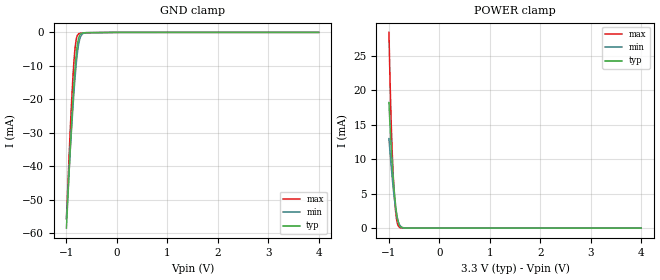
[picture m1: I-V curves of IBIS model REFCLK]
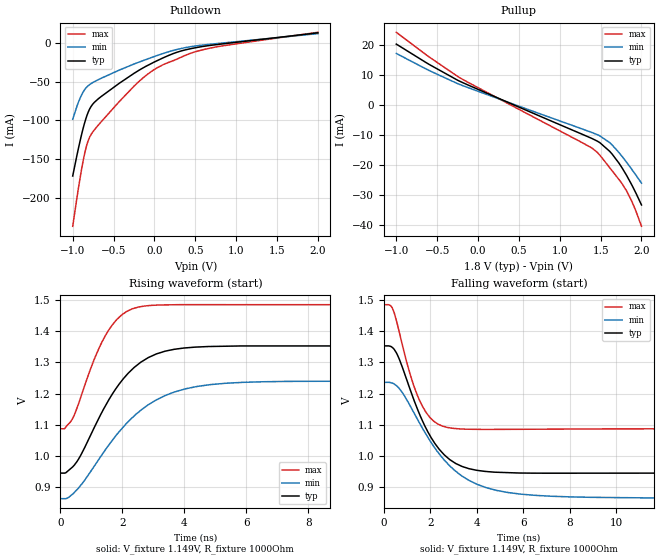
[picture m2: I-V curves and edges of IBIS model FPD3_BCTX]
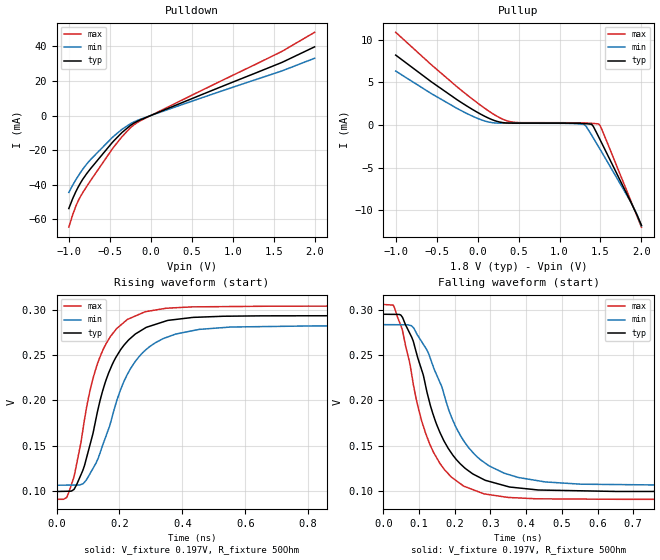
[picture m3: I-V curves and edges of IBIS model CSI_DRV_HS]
|Texas Instruments Incorporated
| Marketing part#   Package-type   #pins
| DS90UB962-Q1   VQFN   64
[IBIS Ver]   4.1
[File name]   ds90ub962q1.ibs
[File Rev]   1.1
[Date]   09/20/2017
[Source]
| Texas Instruments Incorporated.
| 12500 TI Blvd
| Dallas, TX -75243
[Notes]   Revision History:
| Rev 1.2: 09/20/2017
| - Matrix package model added.
| Rev 1.1:  07/22/2016
| - Various signal names modified to reflect the latest datasheet.
| - Various model names modified to reflect I/O character.
| - Unused models removed.
| Rev 1.0: 07/23/2015
| - Initial version of the model
| - Model generated from simulations in TISPICE
| - C_comp although listed in numerical order of value are
|   obtained from varying PVT conditions. For PVT conditions for
|   each specific value refer the buffer description under
|   respective [Model]. IBIS model user is responsible for using
|   appropriate C_comp to simulate for Signal Integrity.
| - Warnings regarding combined Non-monotonicity of various models have been
|   reviewd and considered minor and can be ignored.
| - Model names with a trailing _1p8 contain the model for
|   1.8V operation. Model names with a trailing _3p3 contain the model
|   for 3.3V operation.
[Disclaimer]
| This model is designed as an aid for customers of Texas Instruments.
| TI and its licensors and suppliers make no warranties, either expressed
| or implied, with respect to this  model, including the warranties of
| merchantability or fitness for a particular purpose. The model is
| provided solely on an "as is" basis. The entire risk as to its quality
| and performance is with the customer.
[Copyright]
 (C) Copyright 2015 Texas Instruments Incorporated.All rights reserved.
|   Device
[Component]   DS90UB962-Q1
[Manufacturer]   TI
[Package]  |QFN   64
|   typ   min   max
R_pkg   0   0   0
L_pkg   0   0   0
C_pkg   0   0   0
[Pin]  signal_name   model_name   R_pin   L_pin   C_pin
1   VDD18_P3   POWER   NA   NA   NA
2   VDD18_P2   POWER   NA   NA   NA
3   PDB   PDB   NA   NA   NA
4   TESTEN   IO_LVCMOS   NA   NA   NA
5   REFCLK   REFCLK   NA   NA   NA
6   INTB   IO_OPEN_DRAIN   NA   NA   NA
7   I2C_SDA2   IO_OPEN_DRAIN   NA   NA   NA
8   I2C_SCL2   IO_OPEN_DRAIN   NA   NA   NA
9   GPIO0   IO_LVCMOS   NA   NA   NA
10   GPIO1   IO_LVCMOS   NA   NA   NA
11   I2C_SDA   IO_OPEN_DRAIN   NA   NA   NA
12   I2C_SCL   IO_OPEN_DRAIN   NA   NA   NA
13   VDDL1   POWER   NA   NA   NA
14   GPIO2   IO_LVCMOS   NA   NA   NA
15   GPIO3   IO_LVCMOS   NA   NA   NA
16   VDDIO   POWER   NA   NA   NA
17   GPIO4   IO_LVCMOS   NA   NA   NA
18   GPIO5   IO_LVCMOS   NA   NA   NA
19   GPIO6   IO_LVCMOS   NA   NA   NA
20   GPIO7   IO_LVCMOS   NA   NA   NA
21   VDD_CSI0   POWER   NA   NA   NA
22   CSI0_CLKN   CSI_DRV   NA   NA   NA
23   CSI0_CLKP   CSI_DRV   NA   NA   NA
24   CSI0_D0N   CSI_DRV   NA   NA   NA
25   CSI0_D0P   CSI_DRV   NA   NA   NA
26   CSI0_D1N   CSI_DRV   NA   NA   NA
27   CSI0_D1P   CSI_DRV   NA   NA   NA
28   CSI0_D2N   CSI_DRV   NA   NA   NA
29   CSI0_D2P   CSI_DRV   NA   NA   NA
30   CSI0_D3N   CSI_DRV   NA   NA   NA
31   CSI0_D3P   CSI_DRV   NA   NA   NA
32   VDD18A   POWER   NA   NA   NA
33   VDD_CSI1   POWER   NA   NA   NA
34   CSI1_CLKN   CSI_DRV   NA   NA   NA
35   CSI1_CLKP   CSI_DRV   NA   NA   NA
36   CSI1_D0N   CSI_DRV   NA   NA   NA
37   CSI1_D0P   CSI_DRV   NA   NA   NA
38   CSI1_D1N   CSI_DRV   NA   NA   NA
39   CSI1_D1P   CSI_DRV   NA   NA   NA
40   CSI1_D2N   CSI_DRV   NA   NA   NA
41   CSI1_D2P   CSI_DRV   NA   NA   NA
42   CSI1_D3N   CSI_DRV   NA   NA   NA
43   CSI1_D3P   CSI_DRV   NA   NA   NA
44   VDDL2   POWER   NA   NA   NA
45   MODE   IO_STRAP   NA   NA   NA
46   IDX   IO_STRAP   NA   NA   NA
47   VDD18_P1   POWER   NA   NA   NA
48   VDD18_P0   POWER   NA   NA   NA
49   VDD18_FPD0   POWER   NA   NA   NA
50   RIN0+   FPD3   NA   NA   NA
51   RIN0-   FPD3   NA   NA   NA
52   VDD_FPD1   POWER   NA   NA   NA
53   RIN1+   FPD3   NA   NA   NA
54   RIN1-   FPD3   NA   NA   NA
55   VDD18_FPD1   POWER   NA   NA   NA
56   CMLOUTP   NC   NA   NA   NA
57   CMLOUTN   NC   NA   NA   NA
58   VDD18_FPD2   POWER   NA   NA   NA
59   RIN2+   FPD3   NA   NA   NA
60   RIN2-   FPD3   NA   NA   NA
61   VDD_FPD2   POWER   NA   NA   NA
62   RIN3+   FPD3   NA   NA   NA
63   RIN3-   FPD3   NA   NA   NA
64   VDD18_FPD3   POWER   NA   NA   NA
[Diff Pin]  inv_pin  vdiff  tdelay_typ tdelay_min tdelay_max
23   22   NA   NA   NA   NA
25   24   NA   NA   NA   NA
27   26   NA   NA   NA   NA
29   28   NA   NA   NA   NA
31   30   NA   NA   NA   NA
35   34   NA   NA   NA   NA
37   36   NA   NA   NA   NA
39   38   NA   NA   NA   NA
41   40   NA   NA   NA   NA
43   42   NA   NA   NA   NA
50   51   NA   NA   NA   NA
53   54   NA   NA   NA   NA
59   60   NA   NA   NA   NA
62   63   NA   NA   NA   NA
|   Model Selectors
[Model Selector]  CSI_DRV
CSI_DRV_HS   csi driver in normal mode
CSI_DRV_LP   csi driver in low power mode
[Model Selector]  FPD3
FPD3_RCV   FPD3 buffer in receiver model
FPD3_BCTX   FPD3 buffer in driver model
[Model Selector]  IO_LVCMOS
IO_LVCMOS_1p8  input buffer at 1.8V operation.
IO_LVCMOS_3p3  input buffer at 3.3V operation.
[Define Package Model]  dp90ub60pkg
[Manufacturer]  Unknown
[OEM]  Unknown
[Description]  None
[Number Of Pins]  64
[Pin Numbers]
|Pin Num   Terminal Name
1
2
3
4
5
6
7
8
9
10
11
12
13
14
15
16
17
18
19
20
21
22
23
24
25
26
27
28
29
30
31
32
33
34
35
36
37
38
39
40
41
42
43
44
45
46
47
48
49
50
51
52
53
54
55
56
57
58
59
60
61
62
63
64
[Model Data]
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[End Model Data]
[End Package Model]
| Models and submodels in the file (10): REFCLK (Input), FPD3_BCTX (Output), CSI_DRV_HS (Output), CSI_DRV_LP (Output), FPD3_RCV (Input), IO_LVCMOS_1p8 (I/O), IO_LVCMOS_3p3 (I/O), IO_STRAP (Input), IO_OPEN_DRAIN (I/O_open_drain), PDB (Input)
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|   Model
[Model]   REFCLK
Model_type   Input
Vinl = 0.99
Vinh = 2.31
|   typ   min   max
C_comp   0.217pF   0.155pF   0.285pF
[Voltage Range]   3.3   3   3.6
[Temperature Range]   27   105   -40
[Power Clamp Reference]   3.3   3   3.6
[GND Clamp Reference]   0   0   0
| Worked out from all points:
|   GND clamp passes 1 mA (typ) near -0.74 V on its own axis
|   POWER clamp passes 1 mA (typ) near -0.82 V on its own axis
[GND Clamp]
|   Voltage   I(typ)   I(min)   I(max)
-1V       -58.46mA   -55.76mA   -55.55mA
-930mV    -36.46mA   -36.76mA   -30.93mA
-910mV    -30.68mA   -31.67mA   -24.51mA
-875mV    -21.25mA   -23.26mA   -14.4mA
-850mV    -15.22mA   -17.76mA   -8.48mA
-825mV    -9.978mA   -12.8mA    -4.141mA
-810mV    -7.323mA   -10.17mA   -2.45mA
-785mV    -3.906mA   -6.458mA   -964.5uA
-755mV    -1.549mA   -3.298mA   -398.4uA
-720mV    -501.1uA   -1.299mA   -238.6uA
-615mV    -84.48uA   -95.6uA    -122.5uA
4V        0A         0A         0A
[POWER Clamp]
|   Voltage   I(typ)   I(min)   I(max)
-1V       18.23mA    12.99mA    28.42mA
-980mV    15.09mA    11.12mA    21.96mA
-955mV    11.73mA    8.928mA    15.27mA
-935mV    9.381mA    7.299mA    11.02mA
-910mV    6.809mA    5.441mA    6.923mA
-880mV    4.227mA    3.534mA    3.455mA
-850mV    2.264mA    2.057mA    1.358mA
-830mV    1.348mA    1.339mA    626.9uA
-800mV    532.9uA    639uA      172.3uA
-740mV    64.05uA    118uA      16.27uA
-665mV    7.756uA    15.09uA    5.838uA
4V        0A         0A         0A
|   Model
[Model]   FPD3_BCTX
Model_type   Output
Polarity   Non-Inverting
Vmeas = 1.6
Vref = 1.8
Cref = 1pF
Rref = 50
|   typ   min   max
C_comp   0.938pF   0.681pF   1.119pF
[Voltage Range]   1.8   1.71   1.89
[Temperature Range]   27   105   -40
[Pullup Reference]   1.8   1.71   1.89
[Pulldown Reference]   -0   0   0
[Power Clamp Reference]   1.8   1.71   1.89
[GND Clamp Reference]   0   0   0
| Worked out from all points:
|   slope of the pulldown table from 0 to 0.27 V, typ, clamps not added: 22 ohm
|   slope of the pullup table from 0 to 0.27 V, typ, clamps not added: 84.2 ohm
|   falling waveform, V_fixture 1.149V, R_fixture 1000Ohm: 20-80 % time 1.47ns typ, 2.2ns min, 976ps max; typ from 1.35 V to 0.946 V
|   rising waveform, V_fixture 1.149V, R_fixture 1000Ohm: 20-80 % time 1.47ns typ, 1.91ns min, 987ps max; typ from 0.946 V to 1.35 V
[Pulldown]
|   Voltage   I(typ)   I(min)   I(max)
-1V       -171.7mA   -98.53mA   -236.6mA
-931mV    -136.5mA   -76.76mA   -188.1mA
-877mV    -112.1mA   -64.18mA   -154.7mA
-838mV    -97.47mA   -58.19mA   -135.7mA
-793mV    -85.34mA   -53.79mA   -121.7mA
-649mV    -68.97mA   -45.52mA   -101.5mA
-250mV    -39.27mA   -27.24mA   -55.84mA
-103mV    -30.11mA   -21.43mA   -41.96mA
35mV      -22.8mA    -16.15mA   -31.93mA
248mV     -13.07mA   -9.187mA   -22.14mA
545mV     -5.396mA   -3.33mA    -10.09mA
2V        13.01mA    11.98mA    13.73mA
[Pullup]
|   Voltage   I(typ)   I(min)   I(max)
-1V       20.31mA    17.19mA    24.25mA
-592mV    13.43mA    11.4mA     15.89mA
-223mV    7.882mA    6.809mA    9.073mA
1.262V    -9.676mA   -7.929mA   -12.44mA
1.391V    -11.2mA    -9.211mA   -14.39mA
1.457V    -12.09mA   -9.937mA   -15.81mA
1.49V     -12.62mA   -10.35mA   -16.8mA
1.637V    -16.34mA   -13.28mA   -21.9mA
1.724V    -19.47mA   -15.93mA   -24.93mA
1.814V    -23.4mA    -19.06mA   -28.59mA
1.904V    -27.96mA   -22.41mA   -33.65mA
2V        -33.45mA   -26.17mA   -40.58mA
[Ramp]
R_load = 1000
|   typ   min   max
dV/dt_r   0.243953/1.46588e-09   0.22325/1.90603e-09   0.237963/9.8707e-10
dV/dt_f   0.243821/1.47149e-09   0.22325/2.20309e-09   0.237891/9.7583e-10
[Falling Waveform]
V_fixture = 1.149V
V_fixture_min = 1.054V
V_fixture_max = 1.285V
R_fixture = 1000Ohm
C_fixture = 0F
|   Time   V(typ)   V(min)   V(max)
0s        1.352V     1.236V     1.484V
389.4ps   1.345V     1.232V     1.468V
670.5ps   1.308V     1.215V     1.392V
1.144ns   1.209V     1.158V     1.257V
1.674ns   1.11V      1.087V     1.157V
2.151ns   1.045V     1.03V      1.111V
2.718ns   996.3mV    977.8mV    1.092V
4.025ns   954.3mV    909.4mV    1.085V
5.88ns    945.9mV    878.5mV    1.086V
20ns      946mV      863.8mV    1.087V
[Rising Waveform]
V_fixture = 1.149V
V_fixture_min = 1.054V
V_fixture_max = 1.285V
R_fixture = 1000Ohm
C_fixture = 0F
|   Time   V(typ)   V(min)   V(max)
0s        945.6mV    863.8mV    1.087V
137.5ps   945.6mV    863.8mV    1.088V
422.9ps   968.4mV    881.4mV    1.126V
1.083ns   1.09V      966.8mV    1.308V
1.553ns   1.179V     1.034V     1.402V
1.978ns   1.241V     1.087V     1.452V
2.519ns   1.295V     1.141V     1.477V
3.677ns   1.342V     1.205V     1.484V
5.331ns   1.351V     1.233V     1.484V
20ns      1.352V     1.236V     1.484V
|   Model
[Model]   CSI_DRV_HS
Model_type   Output
Polarity   Non-Inverting
Vmeas = 0.2
Vref = 0.2
Cref = 1pF
Rref = 50
|   typ   min   max
C_comp   0.533pF   0.500pF   0.567pF
[Voltage Range]   1.8   1.71   1.89
[Temperature Range]   27   105   -40
[Pullup Reference]   1.8   1.71   1.89
[Pulldown Reference]   0   0   0
[Power Clamp Reference]   1.8   1.71   1.89
[GND Clamp Reference]   0   0   0
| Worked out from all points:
|   slope of the pulldown table from 0 to 0.27 V, typ, clamps not added: 51.2 ohm
|   slope of the pullup table from 0 to 0.27 V, typ, clamps not added: 240 ohm
|   falling waveform, V_fixture 0.197V, R_fixture 50Ohm: 20-80 % time 106ps typ, 122ps min, 92.5ps max; typ from 0.295 V to 0.1 V
|   rising waveform, V_fixture 0.197V, R_fixture 50Ohm: 20-80 % time 107ps typ, 124ps min, 91.6ps max; typ from 0.1 V to 0.295 V
[Pulldown]
|   Voltage   I(typ)   I(min)   I(max)
-1V       -53.82mA   -44.47mA   -64.6mA
-955mV    -48.34mA   -40.49mA   -57.76mA
-913mV    -43.95mA   -37.09mA   -52.35mA
-877mV    -40.66mA   -34.36mA   -48.58mA
-826mV    -36.62mA   -30.81mA   -44.33mA
-736mV    -30.82mA   -25.57mA   -37.76mA
-454mV    -14.81mA   -12.05mA   -18.38mA
-349mV    -9.736mA   -7.898mA   -12.13mA
-214mV    -4.668mA   -3.904mA   -5.725mA
-40mV     -786.7uA   -671uA     -943.6uA
1.595V    30.62mA    25.72mA    36.98mA
2V        39.75mA    33.16mA    48.16mA
[Pullup]
|   Voltage   I(typ)   I(min)   I(max)
-1V       8.186mA    6.313mA    10.85mA
-562mV    5.036mA    3.655mA    7.03mA
-124mV    2.173mA    1.307mA    3.484mA
104mV     931uA      415.4uA    1.836mA
296mV     288.8uA    201.8uA    718.8uA
464mV     214.7uA    195.7uA    291.1uA
1.301V    155uA      41.19uA    234.5uA
1.397V    22.11uA    -1.28mA    184.5uA
1.481V    -1.468mA   -2.637mA   83.08uA
1.52V     -2.222mA   -3.27mA    -612.7uA
1.868V    -9.009mA   -9.009mA   -8.837mA
2V        -11.77mA   -11.83mA   -11.98mA
[Ramp]
R_load = 50
|   typ   min   max
dV/dt_r   0.117175/1.07008e-10   0.106147/1.24084e-10   0.12875/9.1735e-11
dV/dt_f   0.117128/1.06622e-10   0.10609/1.22337e-10   0.128737/9.23849e-11
[Falling Waveform]
V_fixture = 0.197V
V_fixture_min = 0.195V
V_fixture_max = 0.198V
R_fixture = 50Ohm
C_fixture = 0F
|   Time   V(typ)   V(min)   V(max)
0s        294.8mV    283.3mV    305.5mV
27.18ps   294.7mV    283.3mV    304.9mV
53.33ps   291.5mV    283.2mV    276.9mV
78.72ps   270mV      282.1mV    230mV
106.2ps   234.7mV    265.3mV    178.9mV
157.9ps   165mV      220.2mV    130.8mV
227.9ps   125.5mV    153.7mV    105.1mV
349.1ps   105mV      118.5mV    93.05mV
820.1ps   99.65mV    106.6mV    90.97mV
3.9ns     99.57mV    106.5mV    90.97mV
[Rising Waveform]
V_fixture = 0.197V
V_fixture_min = 0.195V
V_fixture_max = 0.198V
R_fixture = 50Ohm
C_fixture = 0F
|   Time   V(typ)   V(min)   V(max)
0s        99.57mV    106.5mV    90.97mV
33.12ps   99.85mV    106.6mV    93.6mV
65.82ps   108.6mV    106.7mV    133.1mV
110.8ps   156.8mV    121.9mV    217.1mV
157.9ps   222.9mV    161.3mV    262.7mV
201.8ps   254.7mV    210.1mV    282.2mV
236.4ps   268.8mV    235.6mV    290.7mV
349.1ps   287.5mV    269.3mV    301.4mV
820.1ps   293.1mV    282mV      303.7mV
3.9ns     294.9mV    283.4mV    305.5mV
